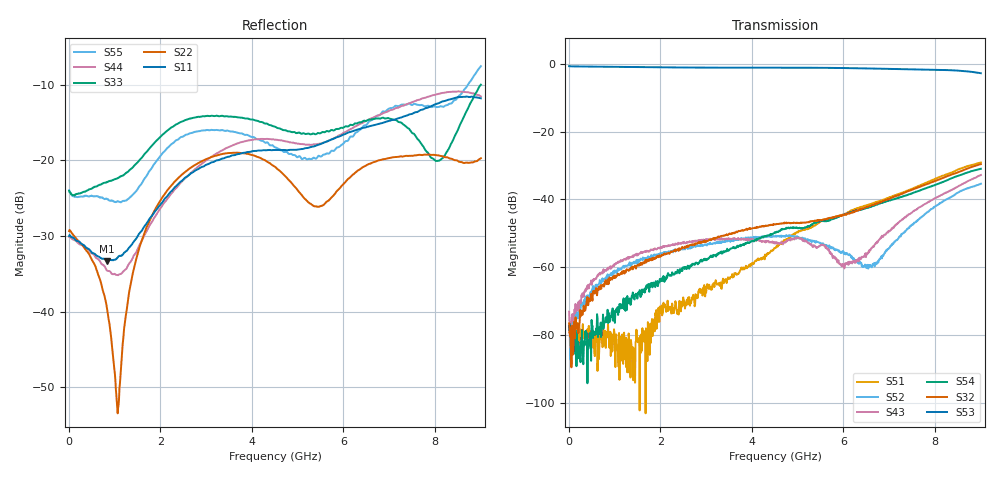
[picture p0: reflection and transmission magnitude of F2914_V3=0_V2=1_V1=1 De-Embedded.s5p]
! Integrated Device Technology
! Corporate Headquarters
! 6024 Silver Creek Valley Road
! San Jose, CA 95138  USA
! Phone:  1-408-284-8200
! Toll Free:  1-800-223-1366
! Webpage:  http://www.idt.com/
! Timing and RF Division
! 515 Groton Road, Suite 102
! Westford, MA 01886-6024
! Device:  F2914
! Description: High Reliability SP4T RF Switch
! Frequency:  0.05 -  8.GHz
! Package:  4x4 mm Thin QFN Plastic Package: 24 pin
! Ports:  5 RF,  5 DC
!  Pin  1  = GND
!  Pin  2  = GND
!  Pin  3  = GND
!  Pin  4  = GND
!  Pin  5  = RF4  =  Port 4
!  Pin  6  = GND
!  Pin  7  = GND
!  Pin  8  = RF3  =  Port 3
!  Pin  9  = GND
!  Pin 10  = GND
!  Pin 11  = RF2  =  Port 2
!  Pin 12  = GND
!  Pin 13  = GND
!  Pin 14  = RF1  =  Port 1
!  Pin 15  = GND
!  Pin 16  = Vcc
!  Pin 17  = V1
!  Pin 18  = V2
!  Pin 19  = V3
!  Pin 20  = VSSext
!  Pin 21  = GND
!  Pin 22  = RFC  =  Port 5
!  Pin 23  = GND
!  Pin 24  = GND
! Voltage:  VDD  =  +3.30 Volts
!  VSSEXT =  0.00 Volts
! Current:  IDD  = 331  uA
! State:  All OFF  RF4 Selected
! V1:  Logic HIGH
! V2:  Logic HIGH
! V3:  Logic LOW
! Data:  The device was measured on the F291x evaluation board which has
!  individual transmission lines to the RF pins.  Data was collected
!  using a calibrated network analyzer.  The input lines were
!  modeled using Automatic Fixture Removal (AFR) from Keysight.
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# Hz S  dB  R 50
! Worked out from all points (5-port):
!   900 points, 10 MHz to 9 GHz, reference 50 ohm
!   strongest paths, dB at 10 MHz, 2.26 GHz, 4.51 GHz, 6.76 GHz, 9 GHz:
!     S53: -0.7, -1.1, -1.2, -1.5, -2.8
!     S32: -76.5, -55.5, -47.3, -41.0, -29.6
!     S54: -78.3, -61.5, -49.7, -41.4, -31.0
!     S43: -73.0, -53.3, -52.6, -52.2, -32.8
!     S52: -77.9, -55.3, -50.9, -58.6, -35.4
!     S51: -79.2, -70.6, -54.3, -40.5, -29.1
!   lowest |S11| = -33.3 dB at 840 MHz (marker M1), VSWR 1.04, Z = 48.6 + j1.56 ohm
!   |S11| at or under -10 dB: start of sweep to end of sweep
